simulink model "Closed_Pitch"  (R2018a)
settings: Solver=ode45  StartTime=0.0  StopTime=80  RelTol=1e-3  EnableMultiTasking=on
InitFcn:
  | init
StopFcn:
  | pl
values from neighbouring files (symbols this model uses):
  Aact = [0, 1; -omg^2, -2*zet*omg]    [init.m]
  Bact = [0; omg^2]    [init.m]
  Cact = [1,0]    [init.m]
  Cza = -0.073    [init.m]
  Czelv = [0.51664,0.51664,0.60478,0.60478,0.06]/100    [init.m]
  d2r = pi/180    (= 0.0174532925199)    [init.m]
  Dact = 0    [init.m]
  Mass = 198.32    [init.m]    (also in lqr_des.m)
  Qbar = 150    [init.m]    (also in lqr_des.m)
  r2d = 180/pi    (= 57.2957795131)    [init.m]    (also in pl.m)
  Sref = 79.069    [init.m]    (also in lqr_des.m)
undefined symbols (not defined in the file or in its folder): Ap, Bp, Cp, Dp, Kmix_qa, Kq

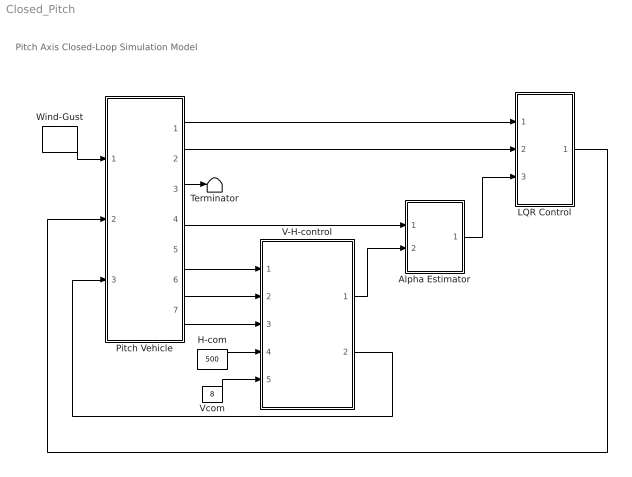
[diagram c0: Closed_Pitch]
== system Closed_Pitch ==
  note: Pitch Axis Closed-Loop Simulation Model
  Alpha Estimator : Subsystem
  H-com : Constant  Value=500
  LQR Control : Subsystem
  Pitch Vehicle : Subsystem
  Terminator : Terminator
  V-H-control : Subsystem
  Vcom : Constant  Value=8
  Wind-Gust : DiscretePulseGenerator  PulseType=Time based  Amplitude=40  Period=100  PulseWidth=5
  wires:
  LQR Control/1(elev) -> Pitch Vehicle/2(elev)
  Pitch Vehicle/1(thet) -> LQR Control/1(thet)
  Pitch Vehicle/2(q) -> LQR Control/2(q)
  Wind-Gust/1 -> Pitch Vehicle/1(Gust)
  Pitch Vehicle/7("Vdot ") -> V-H-control/3(Vdot)
  Pitch Vehicle/6(dH) -> V-H-control/2(dH)
  Pitch Vehicle/4("delv ") -> Alpha Estimator/1(delta)
  V-H-control/2(Throt) -> Pitch Vehicle/3(Thro)
  Alpha Estimator/1(alphat) -> LQR Control/3(alfa)
  V-H-control/1(Zdd-com) -> Alpha Estimator/2(Zdd)
  Pitch Vehicle/5("Az ") -> V-H-control/1(Az)
  H-com/1 -> V-H-control/4(H-comd)
  Vcom/1 -> V-H-control/5(Vcomd)
  Pitch Vehicle/3(alfa) -> Terminator/1

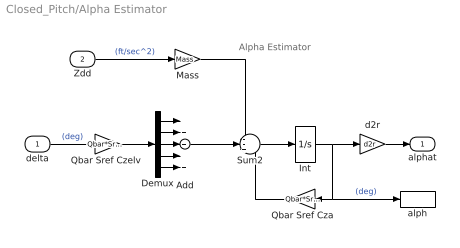
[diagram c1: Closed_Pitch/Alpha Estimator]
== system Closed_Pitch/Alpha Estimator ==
  note: Alpha Estimator
  delta : Inport
  Zdd : Inport  Port=2
  Add : Sum  Inputs=+++++
  Demux : Demux  Outputs=5
  Int : Integrator
  Mass : Gain  Gain=Mass
  Qbar Sref Cza : Gain  Gain=Qbar*Sref*Cza
  "Qbar Sref Czelv " : Gain  Gain=Qbar*Sref*Czelv
  Sum2 : Sum  Inputs=--+
  alph : ToWorkspace  VariableName=alphat  SampleTime=-1
  d2r : Gain  Gain=d2r
  alphat : Outport
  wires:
  d2r/1 -> alphat/1
  Mass/1 -> Sum2/1
  Zdd/1 -> Mass/1  "(ft/sec^2)"
  Qbar Sref Cza/1 -> Sum2/3
  Int/1 -> d2r/1, alph/1, Qbar Sref Cza/1  "(deg)"
  Sum2/1 -> Int/1
  delta/1 -> "Qbar Sref Czelv "/1  "(deg)"
  "Qbar Sref Czelv "/1 -> Demux/1
  Demux/1 -> Add/1
  Demux/2 -> Add/2
  Demux/3 -> Add/3
  Demux/4 -> Add/4
  Demux/5 -> Add/5
  Add/1 -> Sum2/2

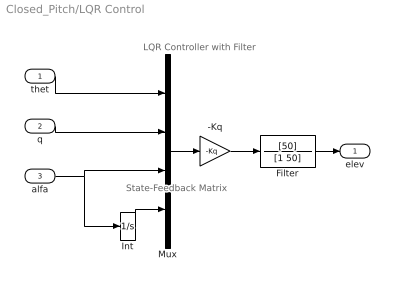
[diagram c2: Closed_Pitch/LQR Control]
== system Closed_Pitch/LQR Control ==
  note: State-Feedback Matrix
  note: LQR Controller with Filter
  thet : Inport
  q : Inport  Port=2
  alfa : Inport  Port=3
  -Kq : Gain  Gain=-Kq  Multiplication=Matrix(K*u)
  Filter : TransferFcn  Numerator=[50]  Denominator=[1 50]
  Int : Integrator
  Mux : Mux
  elev : Outport
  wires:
  alfa/1 -> Int/1, Mux/3
  thet/1 -> Mux/1
  q/1 -> Mux/2
  Filter/1 -> elev/1
  Int/1 -> Mux/4
  Mux/1 -> -Kq/1
  -Kq/1 -> Filter/1

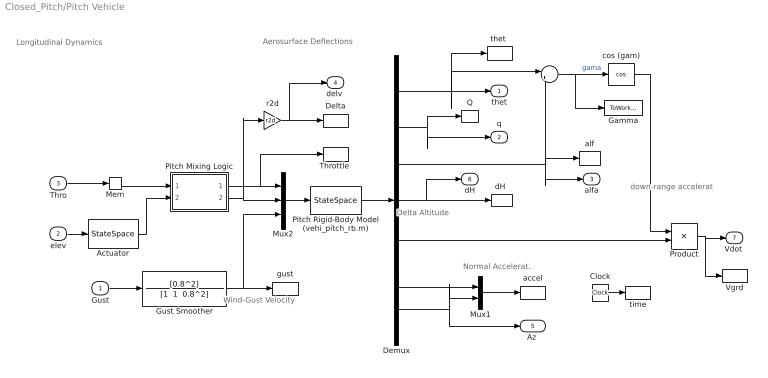
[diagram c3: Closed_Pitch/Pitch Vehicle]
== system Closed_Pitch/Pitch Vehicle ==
  note: Aerosurface Deflections
  note: down-range accelerat
  note: Longitudinal Dynamics
  note: Wind-Gust Velocity
  note: Normal Accelerat.
  note: Delta Altitude
  Gust : Inport
  elev : Inport  Port=2
  Thro : Inport  Port=3
  "    " : Sum  Inputs=|+-
  Actuator : StateSpace  A=Aact  B=Bact  C=Cact  D=Dact  InitialCondition=0
  Clock : Clock
  Delta : ToWorkspace  VariableName=delta  SampleTime=-1
  Demux : Demux  Outputs=7
  Gamma : ToWorkspace  VariableName=gamma  SampleTime=-1
  Gust Smoother : TransferFcn  Numerator=[0.8^2]  Denominator="[1  1  0.8^2]"
  Mem : Memory
  Mux1 : Mux  Inputs=2
  Mux2 : Mux  Inputs=[1, 5, 1]
  Pitch Mixing Logic : Subsystem
  Pitch Rigid-Body Model (vehi_pitch_rb.m) : StateSpace  A=Ap  B=Bp  C=Cp  D=Dp  InitialCondition=0
  Product : Product
  Q : ToWorkspace  VariableName=q  SampleTime=-1
  "Throttle " : ToWorkspace  VariableName=throt  SampleTime=-1
  Vgrd : ToWorkspace  VariableName=Vgrd  SampleTime=-1
  accel : ToWorkspace  VariableName=Accl  SampleTime=-1
  alf : ToWorkspace  VariableName=alfa  SampleTime=-1
  cos (gam) : Trigonometry  Operator=cos
  "dH " : ToWorkspace  VariableName=dH  SampleTime=-1
  gust : ToWorkspace  VariableName=gust  SampleTime=-1
  r2d : Gain  Gain=r2d
  "thet " : ToWorkspace  VariableName=theta  SampleTime=-1
  time : ToWorkspace  VariableName=time  SampleTime=-1
  thet : Outport
  q : Outport  Port=2
  alfa : Outport  Port=3
  "delv " : Outport  Port=4
  "Az " : Outport  Port=5
  dH : Outport  Port=6
  "Vdot " : Outport  Port=7
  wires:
  Pitch Rigid-Body Model (vehi_pitch_rb.m)/1 -> Demux/1
  Mux2/1 -> Pitch Rigid-Body Model (vehi_pitch_rb.m)/1
  Thro/1 -> Mem/1
  Demux/5 -> Product/2
  Demux/4 -> "dH "/1, dH/1
  Gust/1 -> Gust Smoother/1
  elev/1 -> Actuator/1
  Demux/1 -> "thet "/1, thet/1, "    "/1
  Demux/2 -> q/1, Q/1
  Demux/3 -> alf/1, alfa/1, "    "/2
  Demux/6 -> Mux1/1
  Demux/7 -> "Az "/1, Mux1/2
  "    "/1 -> cos (gam)/1, Gamma/1  "gama"
  cos (gam)/1 -> Product/1
  Product/1 -> "Vdot "/1, Vgrd/1
  Gust Smoother/1 -> Mux2/3, gust/1
  Pitch Mixing Logic/1(Thro) -> Mux2/1, "Throttle "/1
  Pitch Mixing Logic/2(delta) -> Mux2/2, r2d/1
  Actuator/1 -> Pitch Mixing Logic/2(delv)
  r2d/1 -> "delv "/1, Delta/1
  Mem/1 -> Pitch Mixing Logic/1(Throt)
  Mux1/1 -> accel/1
  Clock/1 -> time/1

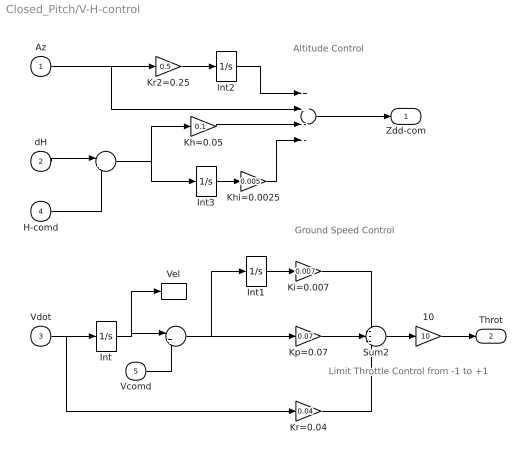
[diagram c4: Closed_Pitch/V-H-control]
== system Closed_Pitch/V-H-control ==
  note: Limit Throttle Control from -1 to +1
  note: Ground Speed Control
  note: Altitude Control
  Az : Inport
  dH : Inport  Port=2
  Vdot : Inport  Port=3
  H-comd : Inport  Port=4
  Vcomd : Inport  Port=5
  " " : Sum  Inputs=|+-
  "  " : Sum  Inputs=++--
  "    " : Sum  Inputs=|+-
  10 : Gain  Gain=10
  Int{,1..3} (4 alike) : Integrator
  Kh=0.05 : Gain  Gain=0.1
  Khi=0.0025 : Gain  Gain=0.005
  Ki=0.007 : Gain  Gain=0.007
  Kp=0.07 : Gain  Gain=0.07
  Kr2=0.25 : Gain  Gain=0.5
  Kr=0.04 : Gain  Gain=0.04
  Sum2 : Sum  Inputs=---
  Vel : ToWorkspace  VariableName=Vel  SampleTime=-1
  Zdd-com : Outport
  Throt : Outport  Port=2
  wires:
  Vdot/1 -> Int/1, Kr=0.04/1
  Sum2/1 -> 10/1
  Kr=0.04/1 -> Sum2/3
  Kp=0.07/1 -> Sum2/2
  Ki=0.007/1 -> Sum2/1
  Int1/1 -> Ki=0.007/1
  Int/1 -> "    "/1, Vel/1
  "    "/1 -> Kp=0.07/1, Int1/1
  Vcomd/1 -> "    "/2
  dH/1 -> " "/1
  H-comd/1 -> " "/2
  Kh=0.05/1 -> "  "/3
  Kr2=0.25/1 -> Int2/1
  Int2/1 -> "  "/1
  Az/1 -> Kr2=0.25/1, "  "/2
  "  "/1 -> Zdd-com/1
  " "/1 -> Kh=0.05/1, Int3/1
  Int3/1 -> Khi=0.0025/1
  Khi=0.0025/1 -> "  "/4
  10/1 -> Throt/1

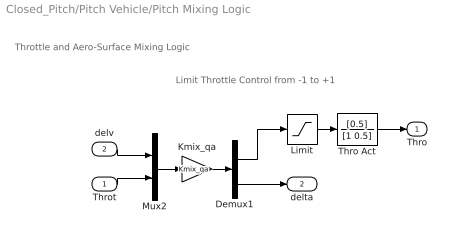
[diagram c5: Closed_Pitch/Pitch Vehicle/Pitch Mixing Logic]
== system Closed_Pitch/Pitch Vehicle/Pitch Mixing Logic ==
  note: Throttle and Aero-Surface Mixing Logic
  note: Limit Throttle Control from -1 to +1
  Throt : Inport
  delv : Inport  Port=2
  Demux1 : Demux  Outputs=[1, 5]
  Kmix_qa : Gain  Gain=Kmix_qa  Multiplication=Matrix(K*u) (u vector)
  Limit : Saturate  UpperLimit=1  LowerLimit=-1
  Mux2 : Mux  Inputs=2
  Thro Act : TransferFcn  Numerator=[0.5]  Denominator=[1 0.5]
  Thro : Outport
  delta : Outport  Port=2
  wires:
  Throt/1 -> Mux2/2
  delv/1 -> Mux2/1
  Demux1/2 -> delta/1
  Demux1/1 -> Limit/1
  Mux2/1 -> Kmix_qa/1
  Kmix_qa/1 -> Demux1/1
  Limit/1 -> Thro Act/1
  Thro Act/1 -> Thro/1
